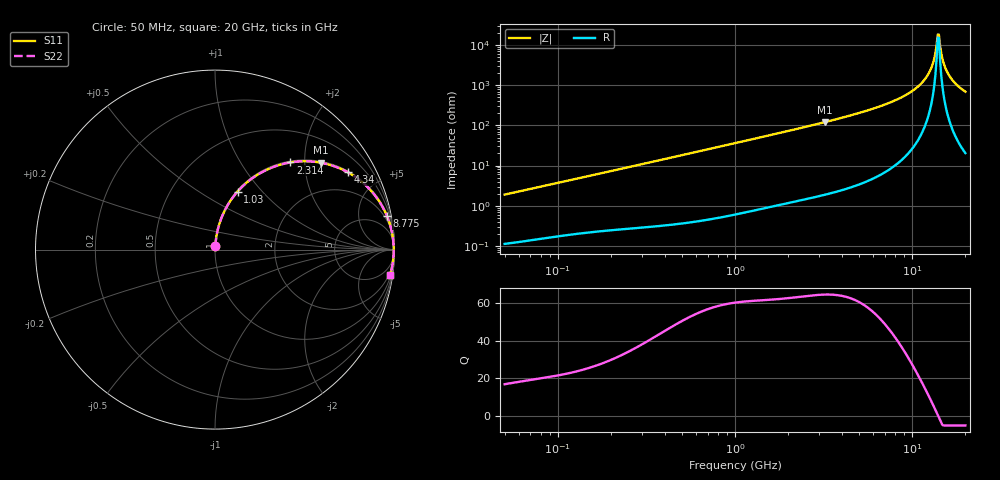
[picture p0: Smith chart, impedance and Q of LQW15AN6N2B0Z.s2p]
!Murata Part Number: LQW15AN6N2B0Z
!These Parameters are Measured in Series Mode Connection
!  o--[Z]--o
!Port1  Port2
!  o-------o
!Freq. Start=50[MHz] Stop=20[GHz], 401[Steps]
# Hz S RI R 50
!Freq.(Hz) S11(Real) S11(Imag) S21(Real) S21(Imag) S12(Real) S12(Imag) S22(Real) S22(Imag)
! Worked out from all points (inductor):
!   401 points, 50 MHz to 20 GHz, reference 50 ohm
!   read as one part in series: L = 5.96 nH near 51.52 MHz
!   highest Q = 64.6 at 3.217 GHz (marker M1), where L = 5.98 nH
!   self-resonance near 13.96 GHz
!   S11 on the Smith chart (normalised r, x): 50 MHz: 1.00, +0.04; 1.03 GHz: 1.01, +0.74; 2.314 GHz: 1.03, +1.70; 4.34 GHz: 1.05, +3.41; 8.775 GHz: 1, +10; 20 GHz: 1, -14
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5e7  0.00146 0.0188  0.9985 -0.0188  0.9985 -0.0188  0.00146 0.0188
1.364002e8  0.00454 0.0498  0.9955 -0.0498  0.9955 -0.0498  0.00454 0.0498
3.721004e8  0.0208 0.1316  0.9792 -0.1316  0.9792 -0.1316  0.0208 0.1316
1e9  0.1196 0.3163  0.8804 -0.3163  0.8804 -0.3163  0.1196 0.3163
1.030411e9  0.1259 0.3236  0.8741 -0.3236  0.8741 -0.3236  0.1259 0.3236
2.313601e9  0.4201 0.4857  0.5799 -0.4857  0.5799 -0.4857  0.4201 0.4857
2.728004e9  0.5052 0.4922  0.4948 -0.4922  0.4948 -0.4922  0.5052 0.4922
3.216634e9  0.5922 0.4837  0.4078 -0.4837  0.4078 -0.4837  0.5922 0.4837
4.34015e9  0.7407 0.4304  0.2593 -0.4304  0.2593 -0.4304  0.7407 0.4304
7.442007e9  0.9261 0.251  0.0739 -0.251  0.0739 -0.251  0.9261 0.251
8.774992e9  0.9582 0.1869  0.0418 -0.1869  0.0418 -0.1869  0.9582 0.1869
1.050288e10  0.9814 0.1159  0.0186 -0.1159  0.0186 -0.1159  0.9814 0.1159
1.201863e10  0.9914 0.0624  0.00864 -0.0624  0.00864 -0.0624  0.9914 0.0624
1.295331e10  0.9943 0.0327  0.00568 -0.0327  0.00568 -0.0327  0.9943 0.0327
1.334722e10  0.995 0.0208  0.005 -0.0208  0.005 -0.0208  0.995 0.0208
1.375312e10  0.9954 0.00886  0.00461 -0.00886  0.00461 -0.00886  0.9954 0.00886
1.396067e10  0.9955 0.0029  0.00452 -0.0029  0.00452 -0.0029  0.9955 0.0029
1.438523e10  0.9954 -0.009  0.00456 0.009  0.00456 0.009  0.9954 -0.009
1.504638e10  0.9948 -0.0269  0.00516 0.0269  0.00516 0.0269  0.9948 -0.0269
1.597544e10  0.993 -0.0507  0.00697 0.0507  0.00697 0.0507  0.993 -0.0507
1.774144e10  0.9871 -0.0924  0.0129 0.0924  0.0129 0.0924  0.9871 -0.0924
2e10  0.9757 -0.1401  0.0243 0.1401  0.0243 0.1401  0.9757 -0.1401
